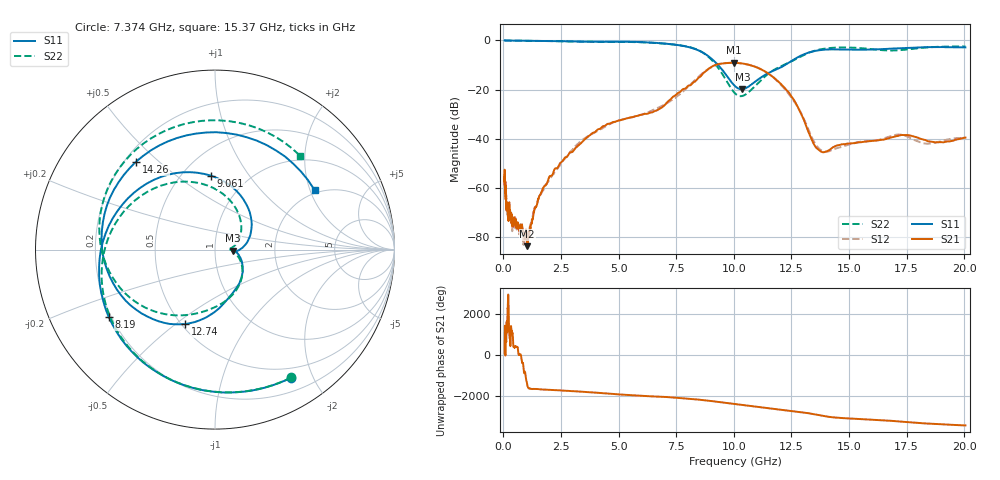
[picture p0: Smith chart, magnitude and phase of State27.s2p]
# Hz S DB R 50
!freq MagS11 AngS11 MagS21 AngS21 MagS12 AngS12 MagS22 AngS22
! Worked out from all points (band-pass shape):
!   1601 points, 50 MHz to 20.05 GHz, reference 50 ohm
!   highest |S21| = -9.11 dB at 9.988 GHz (marker M1); lowest = -83.9 dB at 1.024 GHz (marker M2)
!   |S21| within 3 dB of the highest: 8.838 GHz to 11.25 GHz (2.415 GHz wide, 24 % of centre)
!   lowest |S11| = -19.9 dB at 10.37 GHz (marker M3), VSWR 1.22, Z = 61.2 - j0.81 ohm
!   |S11| at or under -10 dB: 9.315 GHz to 12.23 GHz (2.911 GHz wide, 27 % of centre)
!   |S22| runs from -22.7 to 0.0 dB; largest |S21 - S12| = 0.015
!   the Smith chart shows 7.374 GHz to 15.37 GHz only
!   S11 on the Smith chart (normalised r, x): 7.374 GHz: 0.37, -1.70; 8.19 GHz: 0.19, -0.28; 9.061 GHz: 0.68, +0.68; 12.74 GHz: 0.52, -0.54; 14.26 GHz: 0.24, +0.42; 15.37 GHz: 1.89, +2.15
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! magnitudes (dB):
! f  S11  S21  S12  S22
! 50 MHz  0.0  -58.7  -59.3  0.0
! 90.71 MHz  0.0  -61.9  -58.7  0.0
! 135.9 MHz  0.0  -66.7  -66.9  0.0
! 188.3 MHz  0.0  -67.1  -70.9  0.0
! 218 MHz  0.0  -73.4  -71.9  0.0
! 255.1 MHz  0.0  -66.1  -71.8  0.0
! 369.6 MHz  0.0  -75.7  -74.8  0.0
! 1.005 GHz  -0.1  -80.3  -80.9  -0.1
! 1.024 GHz  -0.1  -83.9  -81.0  -0.1
! 2.722 GHz  -0.3  -47.6  -47.5  -0.4
! 7.374 GHz  -1.6  -22.8  -24.0  -1.6
! 7.402 GHz  -1.6  -22.7  -23.7  -1.7
! 8.19 GHz  -3.1  -17.6  -17.2  -3.0
! 9.061 GHz  -7.7  -10.6  -10.7  -8.2
! 9.988 GHz  -18.0  -9.1  -9.1  -20.9
! 10.37 GHz  -19.9  -9.4  -9.4  -22.6
! 11.69 GHz  -12.4  -14.8  -14.9  -12.3
! 12.74 GHz  -7.0  -26.5  -26.7  -7.3
! 13.58 GHz  -4.2  -43.8  -42.8  -4.0
! 14.26 GHz  -3.6  -43.9  -44.7  -3.0
! 15.37 GHz  -3.8  -41.6  -41.5  -3.0
! 20.05 GHz  -2.8  -39.6  -39.7  -2.4
